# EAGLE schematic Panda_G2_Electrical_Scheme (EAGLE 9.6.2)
AUTHOR: Andrea Maroso; TITLE: Electrical Scheme

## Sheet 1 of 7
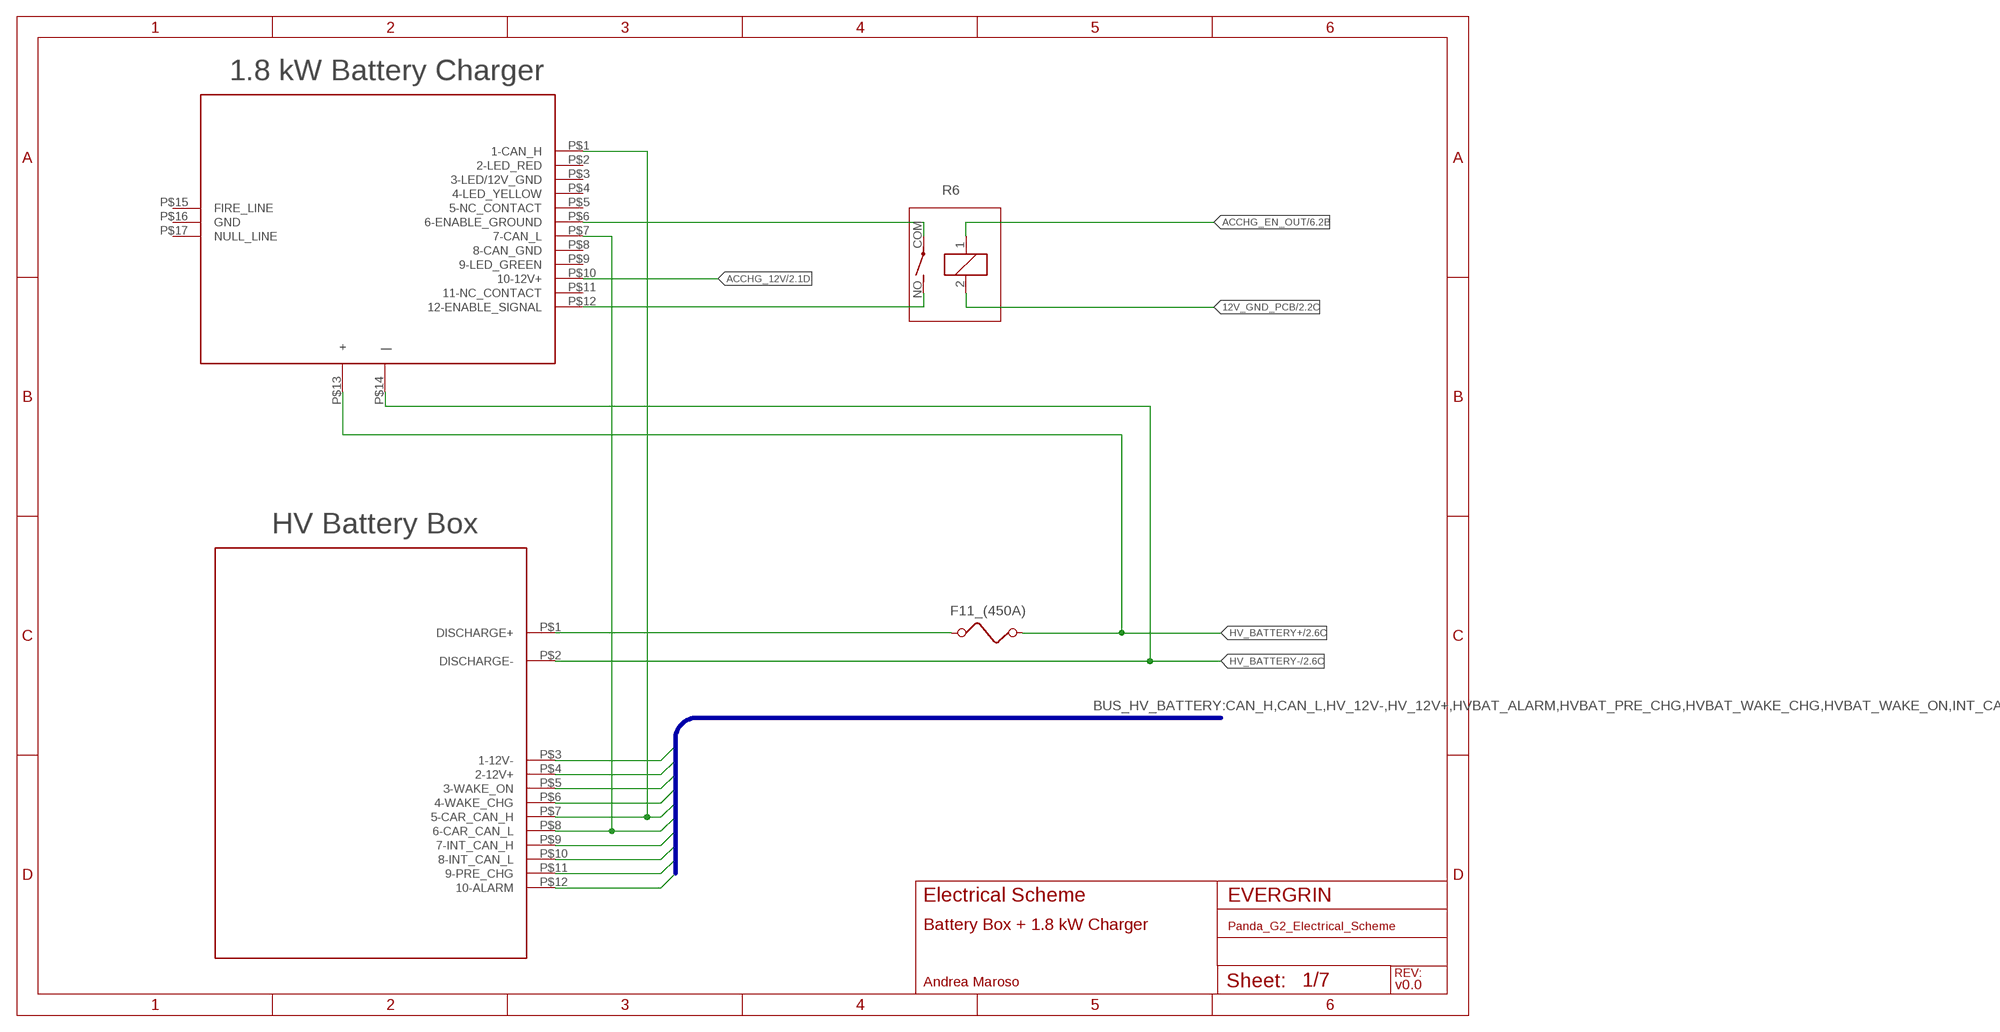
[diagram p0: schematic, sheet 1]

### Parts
F11_(450A)  FUSE  [FUSE]
R6  APF30212A  [APF30212A]
U$1  HV_BATTERY_BOX  [HV_BATTERY_BOX]
U$2  1.8KW_BATTERY_CHARGER  [1.8KW_BATTERY_CHARGER]

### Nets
12V_GND_PCB: R6.2 ; also sheet 2,3,4,5,6,7
ACCHG_12V: U$2.P$10(10-12V+) ; also sheet 2,6
ACCHG_EN_OUT: R6.1 ; also sheet 6
CAN_H: U$1.P$7(5-CAR_CAN_H) U$2.P$1(1-CAN_H) ; also sheet 2,6
CAN_L: U$1.P$8(6-CAR_CAN_L) U$2.P$7(7-CAN_L) ; also sheet 2,6
HV+: F11_(450A).1 U$1.P$1(DISCHARGE+)
HV_12V+: U$1.P$4(2-12V+) ; also sheet 6
HV_12V-: U$1.P$3(1-12V-)
HV_BATTERY+: F11_(450A).2 U$2.P$13(+) ; also sheet 2,4
HV_BATTERY-: U$1.P$2(DISCHARGE-) U$2.P$14(|) ; also sheet 2,4
HVBAT_ALARM: U$1.P$12(10-ALARM) ; also sheet 6
HVBAT_PRE_CHG: U$1.P$11(9-PRE_CHG) ; also sheet 6
HVBAT_WAKE_CHG: U$1.P$6(4-WAKE_CHG) ; also sheet 6
HVBAT_WAKE_ON: U$1.P$5(3-WAKE_ON) ; also sheet 6
INT_CANH: U$1.P$9(7-INT_CAN_H)
INT_CANL: U$1.P$10(8-INT_CAN_L)
N$17: R6.COM(2:P) U$2.P$6(6-ENABLE_GROUND)
N$18: R6.NO(2:S) U$2.P$12(12-ENABLE_SIGNAL)
Unconnected: U$2.P$2(2-LED_RED) U$2.P$3(3-LED/12V_GND) U$2.P$4(4-LED_YELLOW) U$2.P$5(5-NC_CONTACT) U$2.P$8(8-CAN_GND) U$2.P$9(9-LED_GREEN) U$2.P$11(11-NC_CONTACT) U$2.P$15(FIRE_LINE) U$2.P$16(GND) U$2.P$17(NULL_LINE)

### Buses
BUS_HV_BATTERY:CAN_H,CAN_L,HV_12V-,HV_12V+,HVBAT_ALARM,HVBAT_PRE_CHG,HVBAT_WAKE_CHG,HVBAT_WAKE_ON,INT_CANH,INT_CANL

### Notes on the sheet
- Battery Box + 1.8 kW Charger
- v0.0

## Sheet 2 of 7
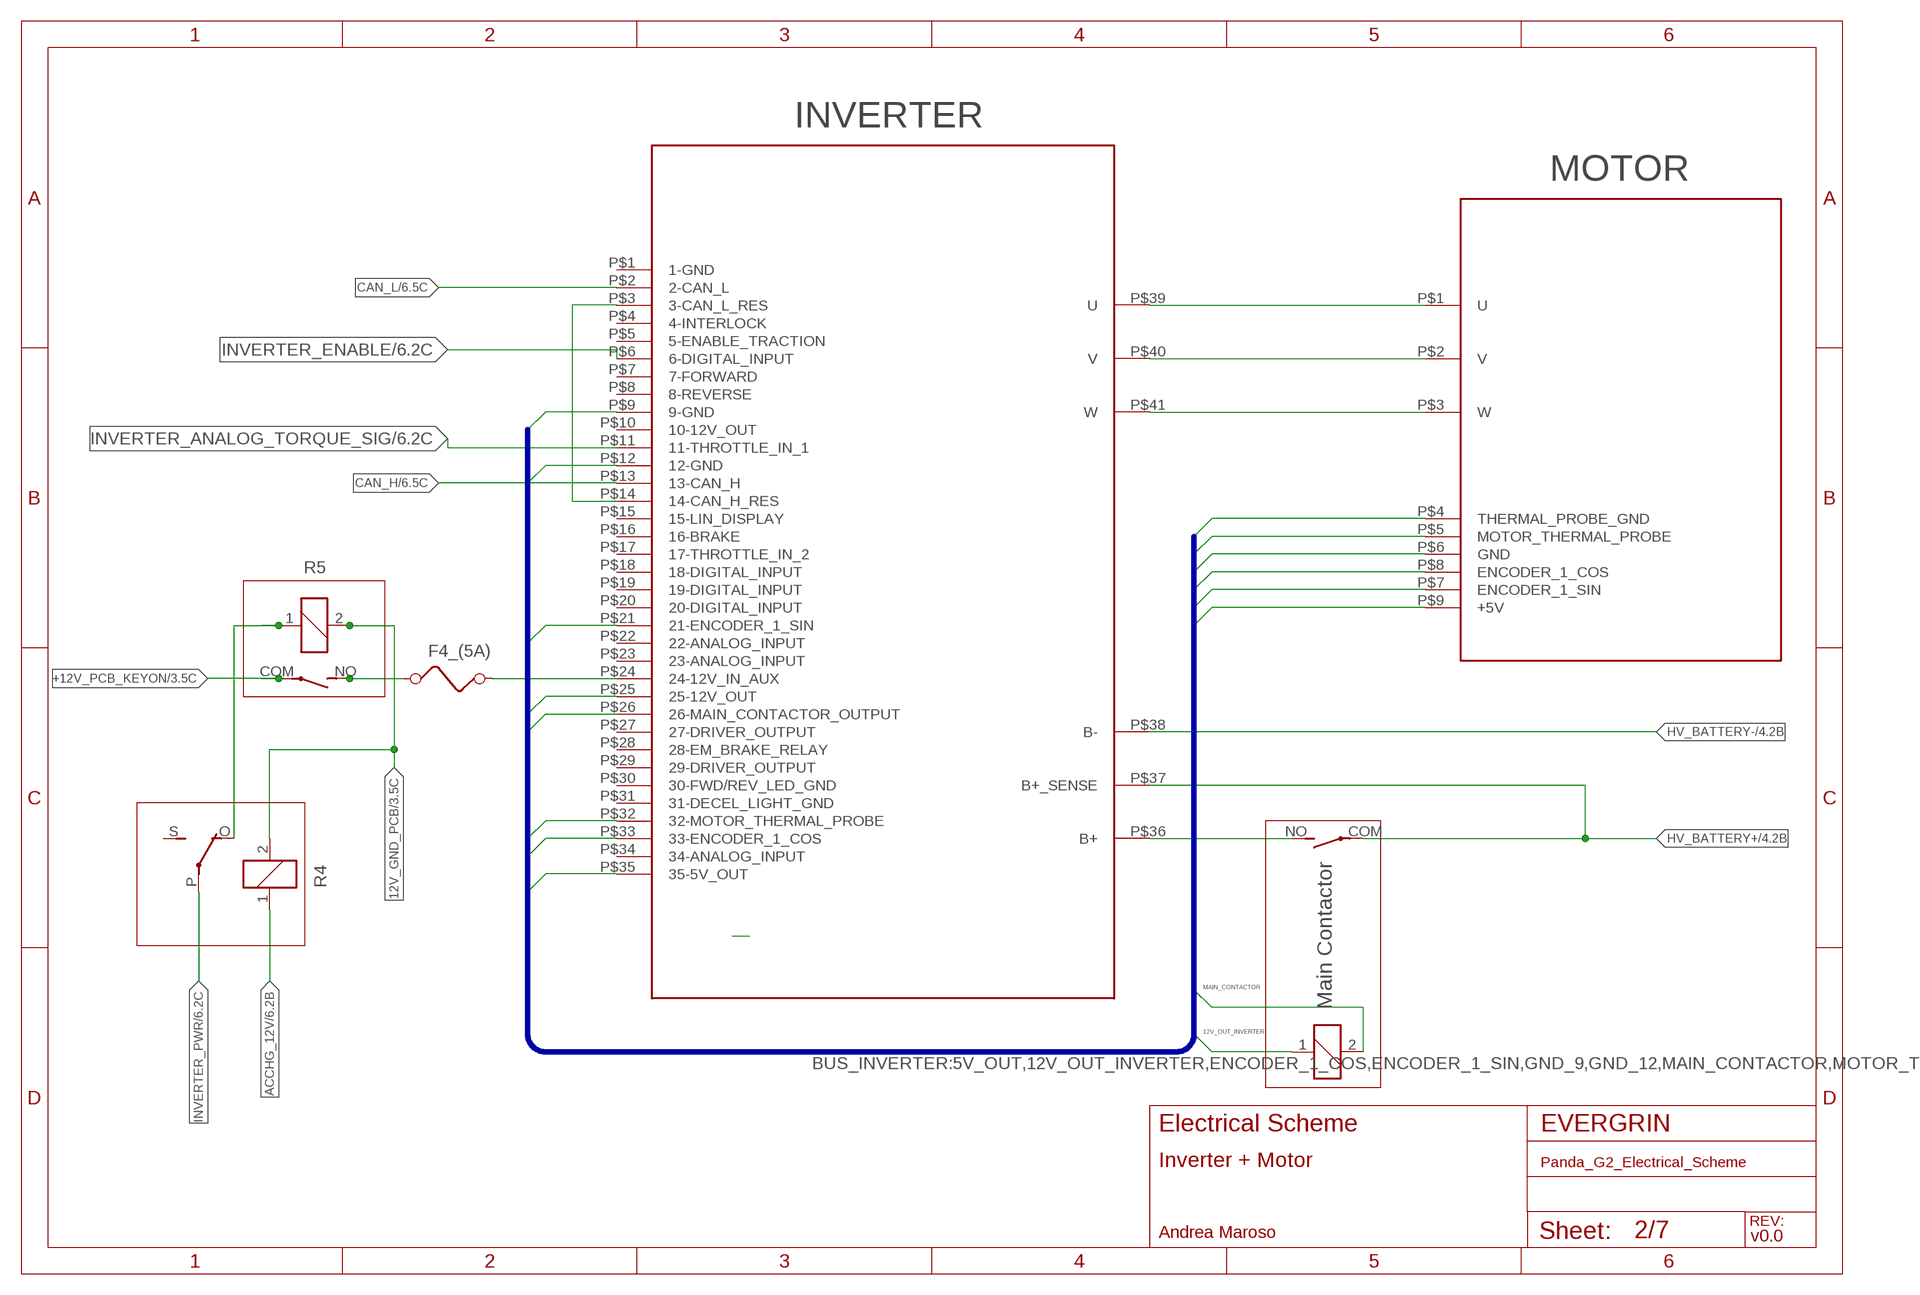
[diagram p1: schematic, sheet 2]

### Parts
F4_(5A)  FUSE  [FUSE]
K1  G5L  [G5LE]
MAIN_CONTACTOR  APF30212A  [APF30212A]
R5  APF30212A  [APF30212A]
U$3  INVERTER  [INVERTER]
U$4  MOTOR  [MOTOR]

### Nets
5V_OUT: U$3.P$35(35-5V_OUT) U$4.P$9(+5V)
12V_GND_PCB: K1.2 R5.2 ; also sheet 1,3,4,5,6,7
12V_OUT_INVERTER: MAIN_CONTACTOR.1 U$3.P$25(25-12V_OUT)
+12V_PCB_KEYON: R5.COM(2:P) ; also sheet 3,5,7
ACCHG_12V: K1.1 ; also sheet 1,6
ACCHG_EN_OUT2: K1.O(2:O) R5.1
CAN_H: U$3.P$13(13-CAN_H) ; also sheet 1,6
CAN_L: U$3.P$2(2-CAN_L) ; also sheet 1,6
ENCODER_1_COS: U$3.P$33(33-ENCODER_1_COS) U$4.P$8(ENCODER_1_COS)
ENCODER_1_SIN: U$3.P$21(21-ENCODER_1_SIN) U$4.P$7(ENCODER_1_SIN)
GND_9: U$3.P$9(9-GND) U$4.P$6(GND)
GND_12: U$3.P$12(12-GND) U$4.P$4(THERMAL_PROBE_GND)
HV_BATTERY+: MAIN_CONTACTOR.COM(2:P) U$3.P$37(B+_SENSE) ; also sheet 1,4
HV_BATTERY-: U$3.P$38(B-) ; also sheet 1,4
INVERTER_ANALOG_TORQUE_SIG: U$3.P$11(11-THROTTLE_IN_1) ; also sheet 6
INVERTER_ENABLE: U$3.P$6(6-DIGITAL_INPUT) ; also sheet 6
INVERTER_PWR: K1.P(2:P) ; also sheet 6
MAIN_CONTACTOR: MAIN_CONTACTOR.2 U$3.P$26(26-MAIN_CONTACTOR_OUTPUT)
MOTOR_THERMAL_PROBE: U$3.P$32(32-MOTOR_THERMAL_PROBE) U$4.P$5(MOTOR_THERMAL_PROBE)
N$1: U$3.P$3(3-CAN_L_RES) U$3.P$14(14-CAN_H_RES)
N$2: U$3.P$39(U) U$4.P$1(U)
N$3: U$3.P$40(V) U$4.P$2(V)
N$4: U$3.P$41(W) U$4.P$3(W)
N$5: MAIN_CONTACTOR.NO(2:S) U$3.P$36(B+)
N$23: F4_(5A).1 R5.NO(2:S)
N$24: F4_(5A).2 U$3.P$24(24-12V_IN_AUX)
Unconnected: K1.S(2:S) U$3.P$1(1-GND) U$3.P$4(4-INTERLOCK) U$3.P$5(5-ENABLE_TRACTION) U$3.P$7(7-FORWARD) U$3.P$8(8-REVERSE) U$3.P$10(10-12V_OUT) U$3.P$15(15-LIN_DISPLAY) U$3.P$16(16-BRAKE) U$3.P$17(17-THROTTLE_IN_2) U$3.P$18(18-DIGITAL_INPUT) U$3.P$19(19-DIGITAL_INPUT) U$3.P$20(20-DIGITAL_INPUT) U$3.P$22(22-ANALOG_INPUT) U$3.P$23(23-ANALOG_INPUT) U$3.P$27(27-DRIVER_OUTPUT) U$3.P$28(28-EM_BRAKE_RELAY) U$3.P$29(29-DRIVER_OUTPUT) U$3.P$30(30-FWD/REV_LED_GND) U$3.P$31(31-DECEL_LIGHT_GND) U$3.P$34(34-ANALOG_INPUT)

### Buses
BUS_INVERTER:5V_OUT,12V_OUT_INVERTER,ENCODER_1_COS,ENCODER_1_SIN,GND_9,GND_12,MAIN_CONTACTOR,MOTOR_THERMAL_PROBE

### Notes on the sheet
- R4 | Main Contactor
- Inverter + Motor
- v0.0

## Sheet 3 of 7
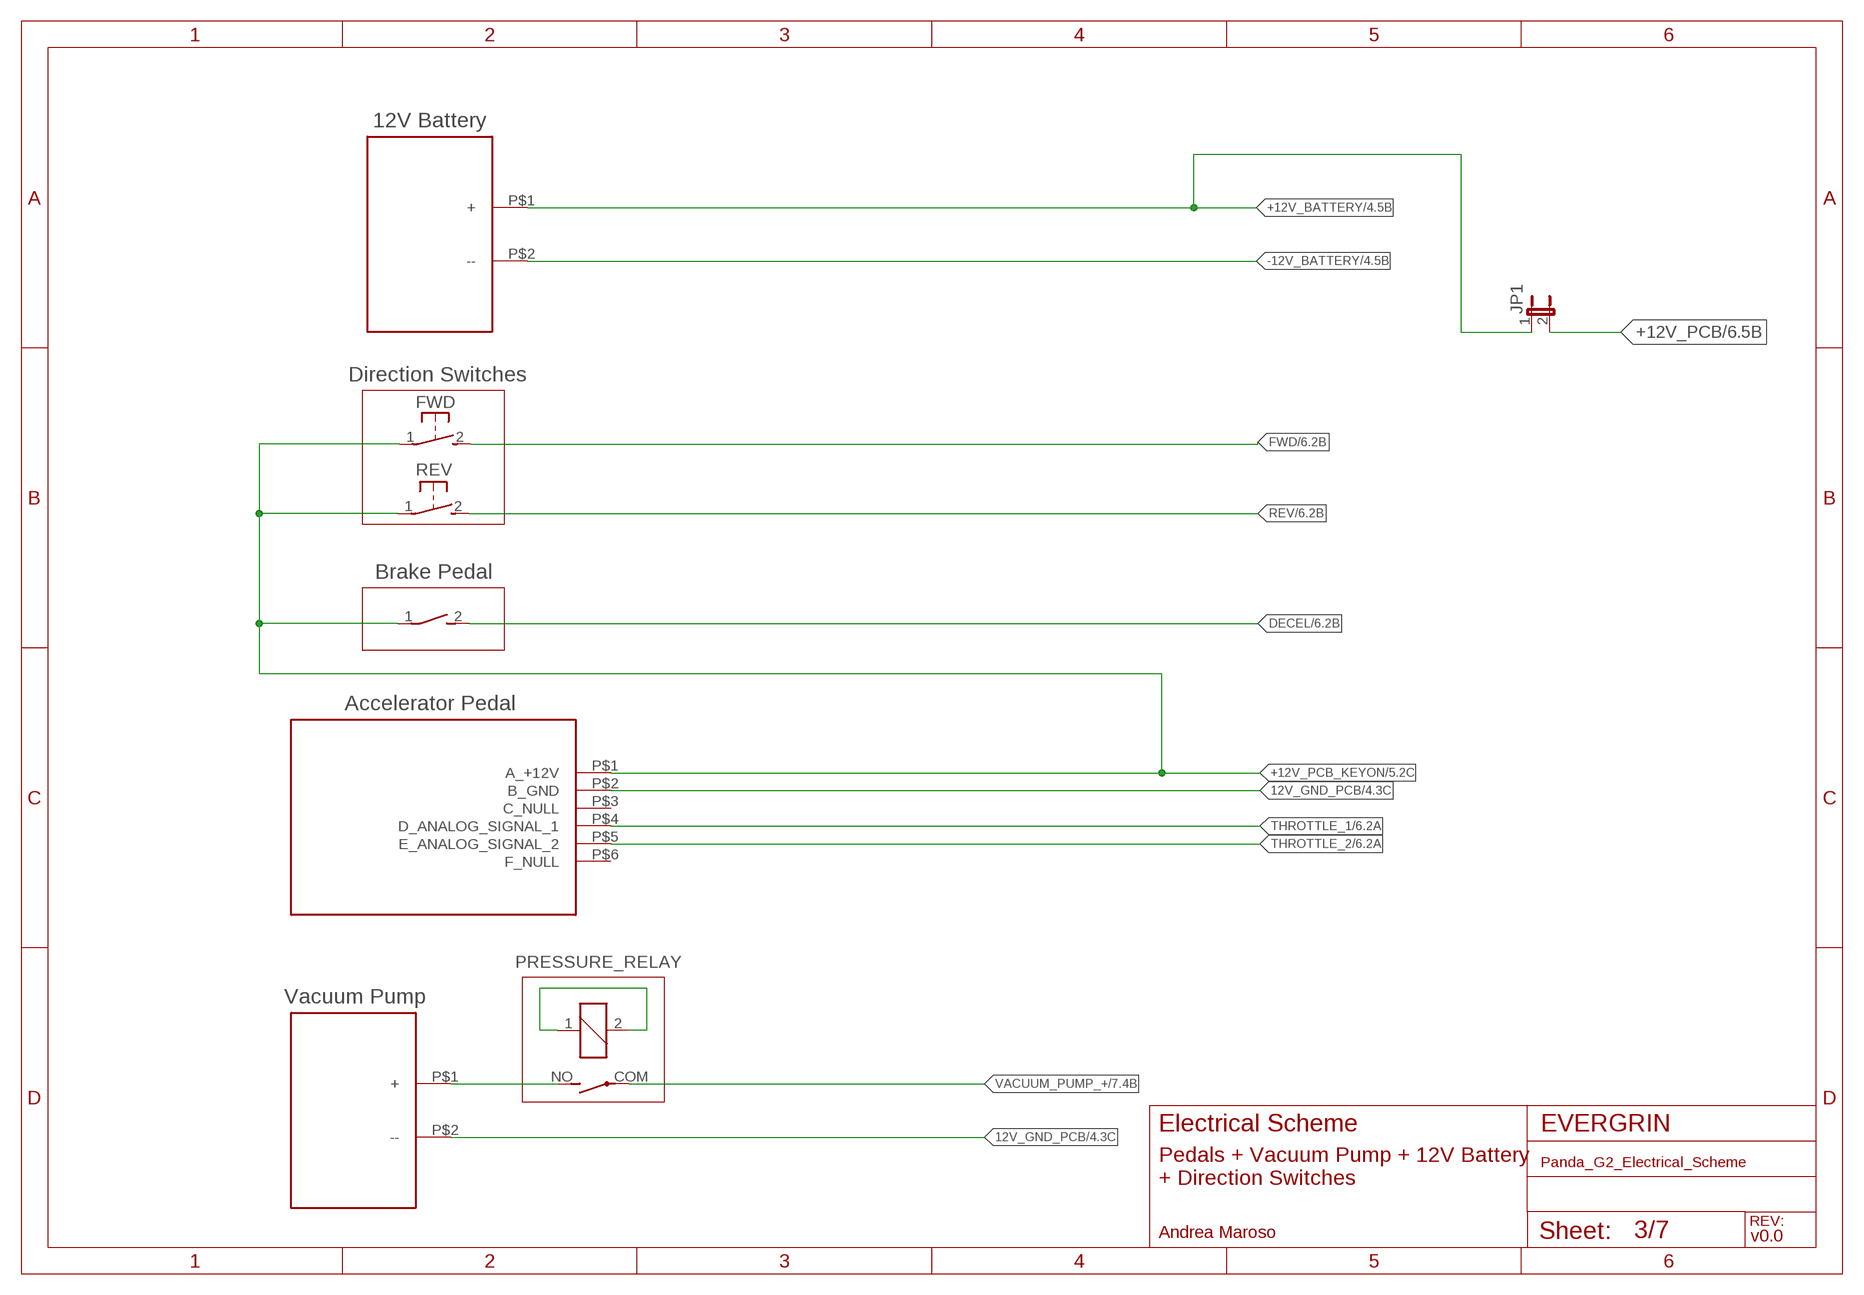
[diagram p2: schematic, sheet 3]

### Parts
JP1  JP1E  [JP1]
PRESSURE_RELAY  APF30212A  [APF30212A]
S1  31-XX  [B3F-31XX]
S2  31-XX  [B3F-31XX]
S4  DS01E  [DS-01]
U$5  12V_BATTERY  [12V_BATTERY]
U$6  ACC_PEDAL  [ACC_PEDAL]
U$7  VACUUM_PUMP  [VACUUM_PUMP]

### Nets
12V_GND_PCB: U$6.P$2(B_GND) U$7.P$2(--) ; also sheet 1,2,4,5,6,7
+12V_BATTERY: JP1.1 U$5.P$1(+) ; also sheet 4,6
+12V_PCB: JP1.2 ; also sheet 6,7
+12V_PCB_KEYON: S1.1(P) S2.1(P) S4.1 U$6.P$1(A_+12V) ; also sheet 2,5,7
-12V_BATTERY: U$5.P$2(--) ; also sheet 4
DECEL: S4.2 ; also sheet 6
FWD: S1.2(S) ; also sheet 6
N$7: PRESSURE_RELAY.1 PRESSURE_RELAY.2
REV: S2.2(S) ; also sheet 6
THROTTLE_1: U$6.P$4(D_ANALOG_SIGNAL_1) ; also sheet 6
THROTTLE_2: U$6.P$5(E_ANALOG_SIGNAL_2) ; also sheet 6
VACUUM_PUMP_+: PRESSURE_RELAY.COM(2:P) PRESSURE_RELAY.NO(2:S) U$7.P$1(+) ; also sheet 7
Unconnected: U$6.P$3(C_NULL) U$6.P$6(F_NULL)

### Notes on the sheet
- Direction Switches
- FWD
- REV
- Brake Pedal
- Pedals + Vacuum Pump + 12V Battery
  + Direction Switches
- v0.0

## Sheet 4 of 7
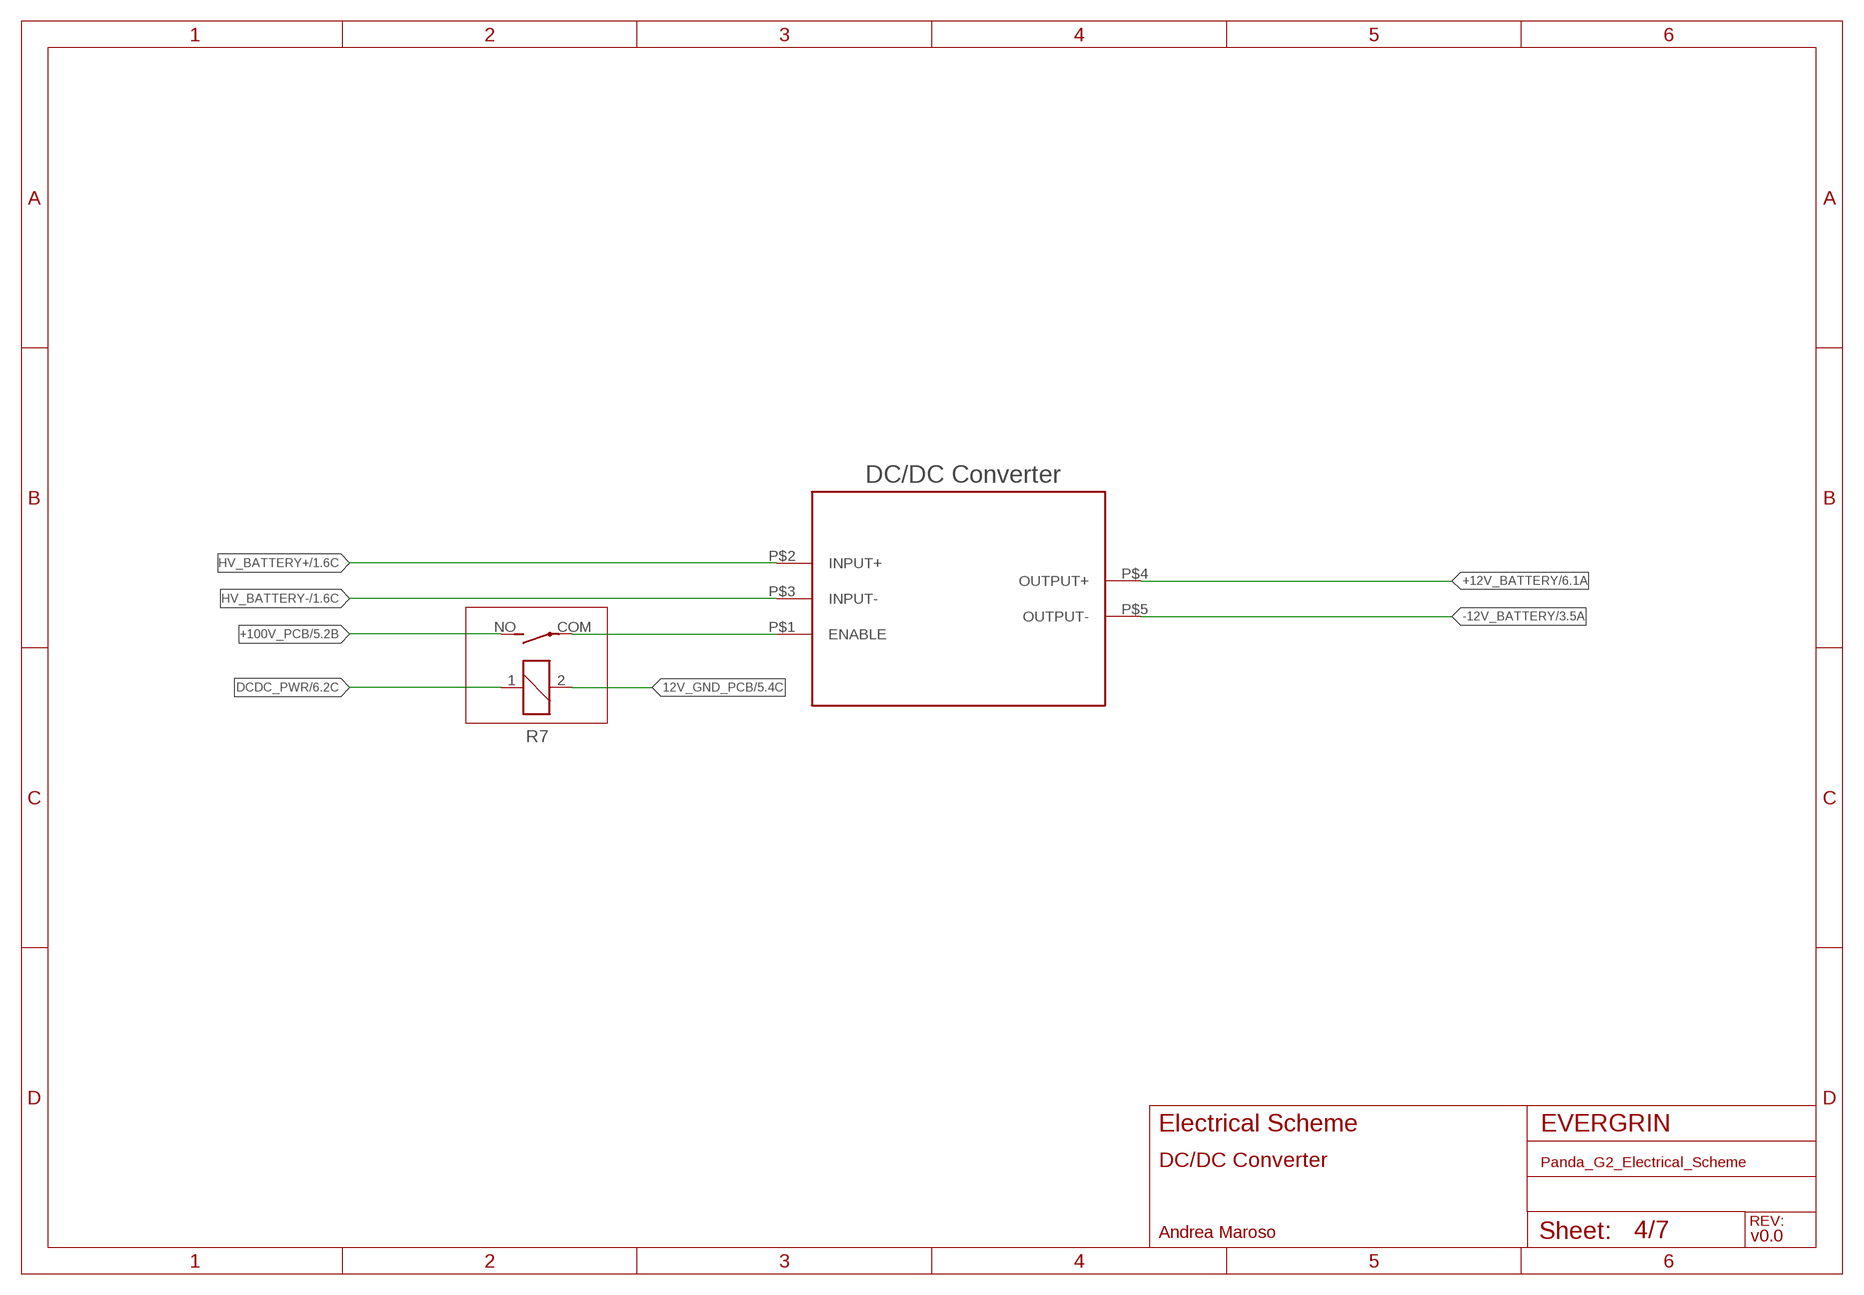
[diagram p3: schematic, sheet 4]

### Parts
R7  APF30212A  [APF30212A]
U$8  DC/DC  [DC/DC]

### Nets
12V_GND_PCB: R7.2 ; also sheet 1,2,3,5,6,7
+12V_BATTERY: U$8.P$4(OUTPUT+) ; also sheet 3,6
+100V_PCB: R7.NO(2:S) ; also sheet 5
-12V_BATTERY: U$8.P$5(OUTPUT-) ; also sheet 3
DCDC_PWR: R7.1 ; also sheet 6
HV_BATTERY+: U$8.P$2(INPUT+) ; also sheet 1,2
HV_BATTERY-: U$8.P$3(INPUT-) ; also sheet 1,2
N$6: R7.COM(2:P) U$8.P$1(ENABLE)

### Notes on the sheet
- DC/DC Converter
- v0.0

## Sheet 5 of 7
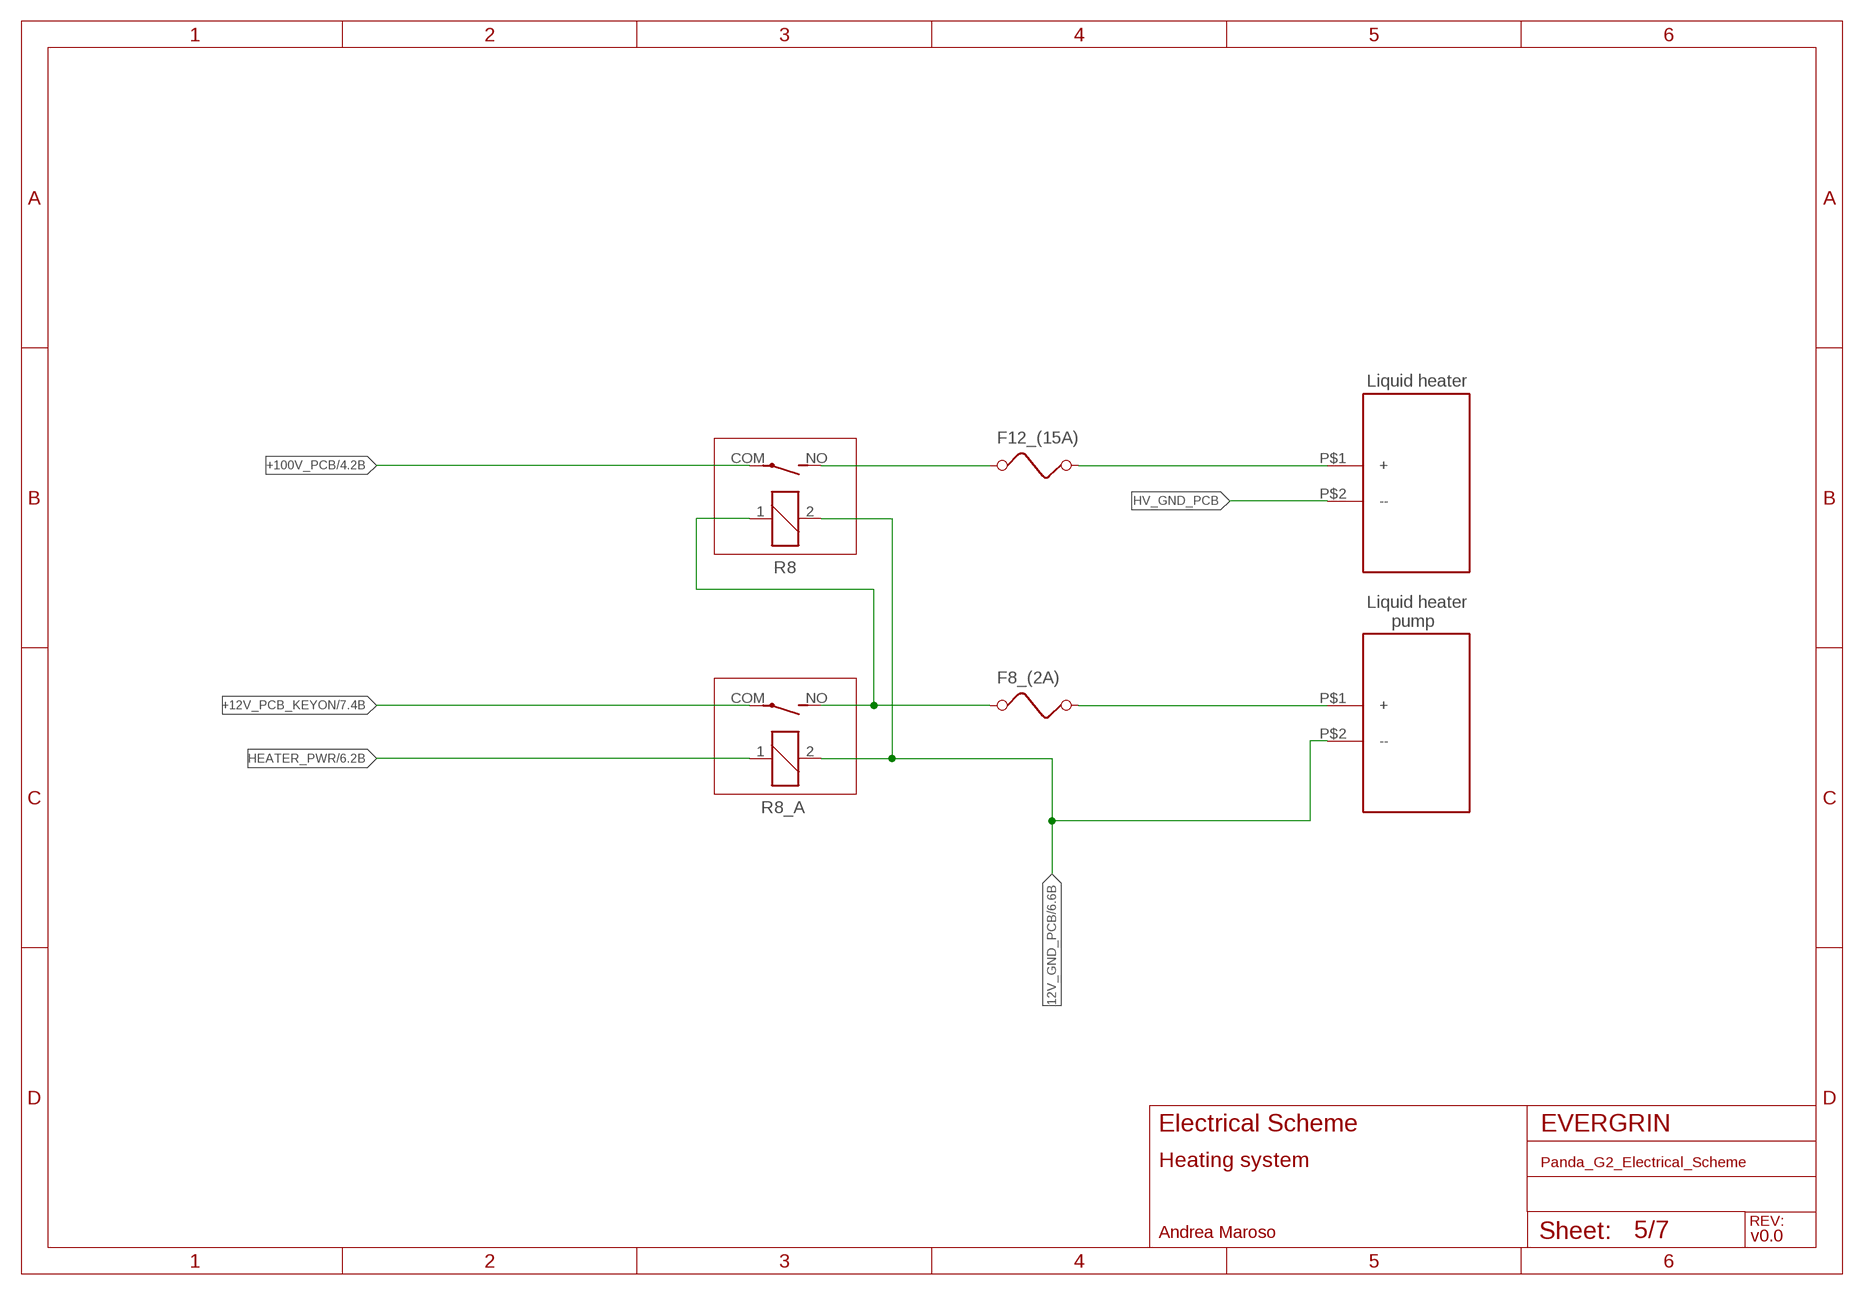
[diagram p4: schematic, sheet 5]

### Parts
F8_(2A)  FUSE  [FUSE]
F12_(15A)  FUSE  [FUSE]
R8  APF30212A  [APF30212A]
R8_A  APF30212A  [APF30212A]
U$9  LIQUID_HEATER  [LIQUID_HEATER]
U$10  LIQUID_HEATER_PUMP  [LIQUID_HEATER_PUMP]

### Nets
12V_GND_PCB: R8.2 R8_A.2 U$10.P$2(--) ; also sheet 1,2,3,4,6,7
+12V_PCB_KEYON: R8_A.COM(2:P) ; also sheet 2,3,7
+100V_PCB: R8.COM(2:P) ; also sheet 4
HEATER_PWR: R8_A.1 ; also sheet 6
HV_GND_PCB: U$9.P$2(--)
N$8: F12_(15A).1 R8.NO(2:S)
N$9: F12_(15A).2 U$9.P$1(+)
N$11: F8_(2A).1 R8.1 R8_A.NO(2:S)
N$12: F8_(2A).2 U$10.P$1(+)

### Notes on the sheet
- Heating system
- v0.0

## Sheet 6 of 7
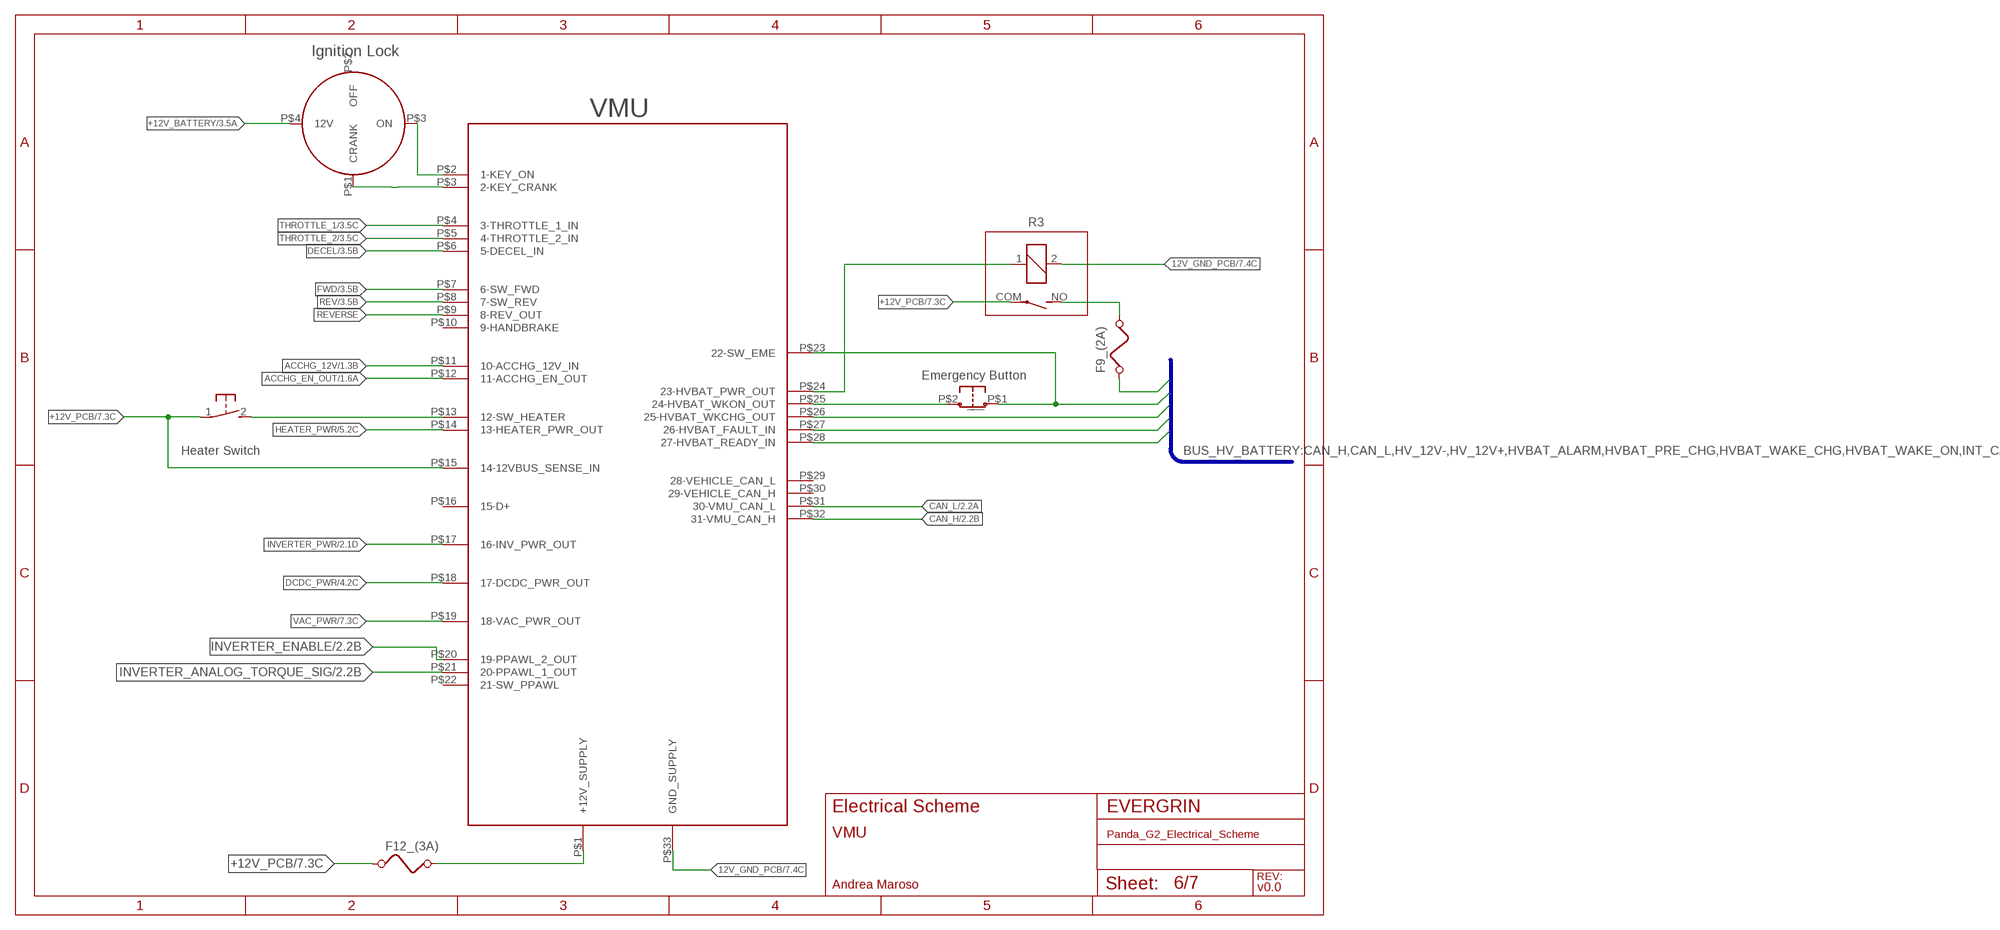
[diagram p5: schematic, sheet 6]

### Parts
F9_(2A)  FUSE  [FUSE]
F12_(3A)  FUSE  [FUSE]
R3  APF30212A  [APF30212A]
S5  31-XX  [B3F-31XX]
U$11  VMU  [VMU]
U$12  IGNITION_LOCK  [IGNITION_LOCK]
U$13  EMERGENCY_BUTTON  [EMERGENCY_BUTTON]

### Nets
12V_GND_PCB: R3.2 U$11.P$33(GND_SUPPLY) ; also sheet 1,2,3,4,5,7
+12V_BATTERY: U$12.P$4(12V) ; also sheet 3,4
+12V_PCB: F12_(3A).1 R3.COM(2:P) S5.1(P) U$11.P$15(14-12VBUS_SENSE_IN) ; also sheet 3,7
ACCHG_12V: U$11.P$11(10-ACCHG_12V_IN) ; also sheet 1,2
ACCHG_EN_OUT: U$11.P$12(11-ACCHG_EN_OUT) ; also sheet 1
CAN_H: U$11.P$32(31-VMU_CAN_H) ; also sheet 1,2
CAN_L: U$11.P$31(30-VMU_CAN_L) ; also sheet 1,2
DCDC_PWR: U$11.P$18(17-DCDC_PWR_OUT) ; also sheet 4
DECEL: U$11.P$6(5-DECEL_IN) ; also sheet 3
FWD: U$11.P$7(6-SW_FWD) ; also sheet 3
HEATER_PWR: U$11.P$14(13-HEATER_PWR_OUT) ; also sheet 5
HV_12V+: F9_(2A).2 ; also sheet 1
HVBAT_ALARM: U$11.P$27(26-HVBAT_FAULT_IN) ; also sheet 1
HVBAT_PRE_CHG: U$11.P$28(27-HVBAT_READY_IN) ; also sheet 1
HVBAT_WAKE_CHG: U$11.P$26(25-HVBAT_WKCHG_OUT) ; also sheet 1
HVBAT_WAKE_ON: U$11.P$23(22-SW_EME) U$13.P$1(_) ; also sheet 1
INVERTER_ANALOG_TORQUE_SIG: U$11.P$21(20-PPAWL_1_OUT) ; also sheet 2
INVERTER_ENABLE: U$11.P$20(19-PPAWL_2_OUT) ; also sheet 2
INVERTER_PWR: U$11.P$17(16-INV_PWR_OUT) ; also sheet 2
KEY_CRANK: U$11.P$3(2-KEY_CRANK) U$12.P$1(CRANK)
KEY_ON: U$11.P$2(1-KEY_ON) U$12.P$3(ON) ; also sheet 7
N$13: U$11.P$25(24-HVBAT_WKON_OUT) U$13.P$2(__)
N$14: F12_(3A).2 U$11.P$1(+12V_SUPPLY)
N$15: R3.1 U$11.P$24(23-HVBAT_PWR_OUT)
N$16: F9_(2A).1 R3.NO(2:S)
N$19: S5.2(S) U$11.P$13(12-SW_HEATER)
REV: U$11.P$8(7-SW_REV) ; also sheet 3
REVERSE: U$11.P$9(8-REV_OUT)
THROTTLE_1: U$11.P$4(3-THROTTLE_1_IN) ; also sheet 3
THROTTLE_2: U$11.P$5(4-THROTTLE_2_IN) ; also sheet 3
VAC_PWR: U$11.P$19(18-VAC_PWR_OUT) ; also sheet 7
Unconnected: U$11.P$10(9-HANDBRAKE) U$11.P$16(15-D+) U$11.P$22(21-SW_PPAWL) U$11.P$29(28-VEHICLE_CAN_L) U$11.P$30(29-VEHICLE_CAN_H) U$12.P$2(OFF)

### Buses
BUS_HV_BATTERY:CAN_H,CAN_L,HV_12V-,HV_12V+,HVBAT_ALARM,HVBAT_PRE_CHG,HVBAT_WAKE_CHG,HVBAT_WAKE_ON,INT_CANH,INT_CANL

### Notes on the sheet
- Heater Switch
- VMU
- v0.0

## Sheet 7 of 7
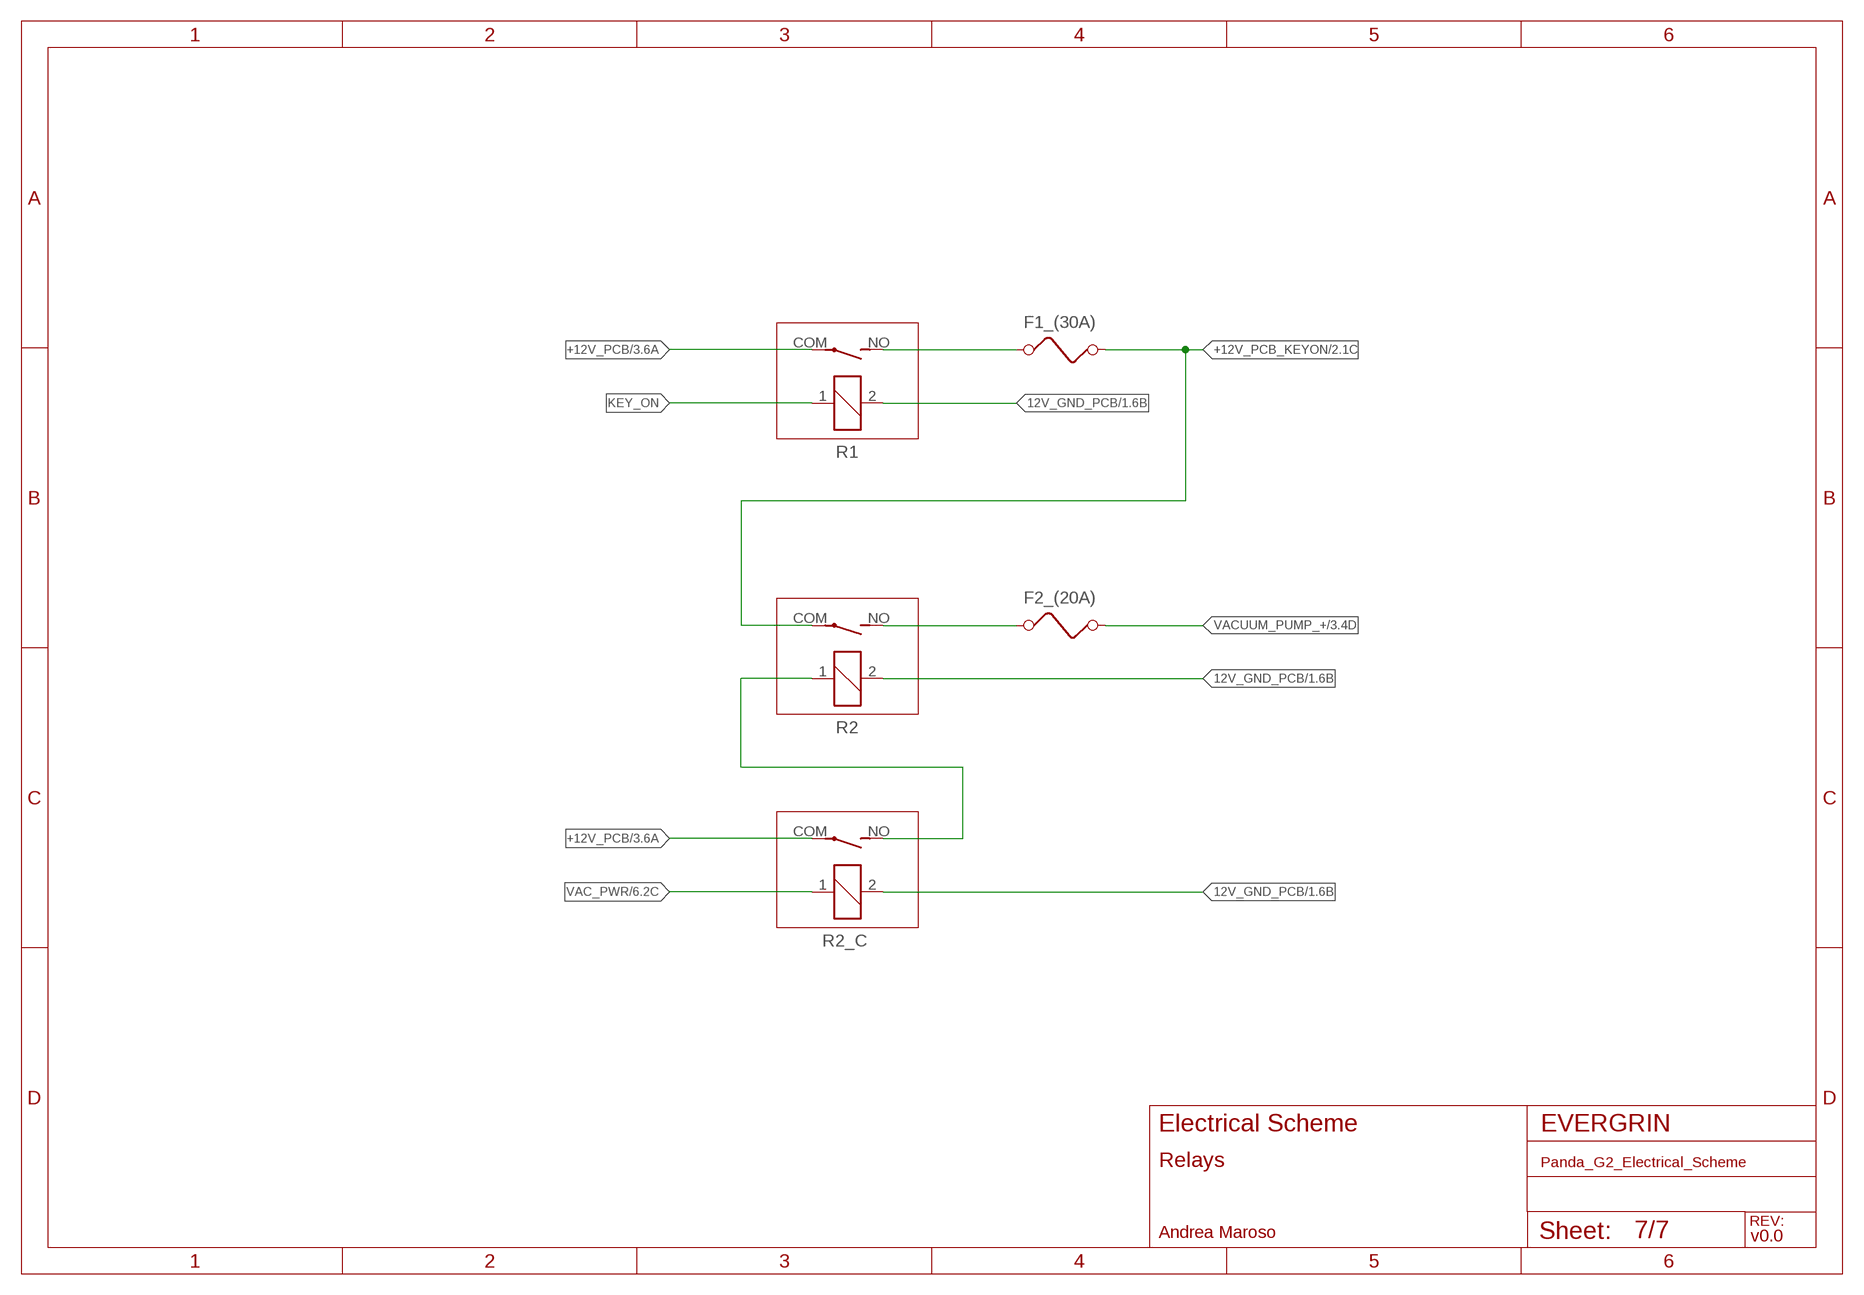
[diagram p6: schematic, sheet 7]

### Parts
F1_(30A)  FUSE  [FUSE]
F2_(20A)  FUSE  [FUSE]
R1  APF30212A  [APF30212A]
R2  APF30212A  [APF30212A]
R2_C  APF30212A  [APF30212A]

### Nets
12V_GND_PCB: R1.2 R2.2 R2_C.2 ; also sheet 1,2,3,4,5,6
+12V_PCB: R1.COM(2:P) R2_C.COM(2:P) ; also sheet 3,6
+12V_PCB_KEYON: F1_(30A).2 R2.COM(2:P) ; also sheet 2,3,5
KEY_ON: R1.1 ; also sheet 6
N$10: F2_(20A).1 R2.NO(2:S)
N$20: F1_(30A).1 R1.NO(2:S)
N$22: R2.1 R2_C.NO(2:S)
VAC_PWR: R2_C.1 ; also sheet 6
VACUUM_PUMP_+: F2_(20A).2 ; also sheet 3

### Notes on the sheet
- Relays
- v0.0

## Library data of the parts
F1_(30A) F2_(20A) F4_(5A) F8_(2A) F9_(2A) F11_(450A) F12_(3A) F12_(15A) = special:FUSE: FUSE
JP1 = jumper:JP1E: JUMPER
K1 = relay:G5L: RELAY 1 x switch, 10 A/120 V AC, 8 A/30 V ADC, Omron; OC_FARNELL: unknown; OC_NEWARK: unknown
MAIN_CONTACTOR PRESSURE_RELAY R1 R2 R2_C R3 R5-R8 R8_A = relay:APF30212A: Compliant with European standards 1a/1c 6A Slim power relays Source: Data sheet; OC_FARNELL: unknown
S1 S2 S5 = switch-omron:31-XX: OMRON SWITCH; MPN: B3F-3100; OC_FARNELL: 959704; OC_NEWARK: 36M3582
S4 = switch-dil:DS01E: DIL/CODE SWITCH; OC_FARNELL: unknown; OC_NEWARK: unknown
U$1 = EVERGRIN_Panda_G2:HV_BATTERY_BOX: HV battery box
U$2 = EVERGRIN_Panda_G2:1.8KW_BATTERY_CHARGER: 1.8 kW battery charger
U$3 = EVERGRIN_Panda_G2:INVERTER: Inverter
U$4 = EVERGRIN_Panda_G2:MOTOR: Motor
U$5 = EVERGRIN_Panda_G2:12V_BATTERY: 12 V battery
U$6 = EVERGRIN_Panda_G2:ACC_PEDAL: Accelerator pedal
U$7 = EVERGRIN_Panda_G2:VACUUM_PUMP
U$8 = EVERGRIN_Panda_G2:DC/DC
U$9 = EVERGRIN_Panda_G2:LIQUID_HEATER: Liquid Heater
U$10 = EVERGRIN_Panda_G2:LIQUID_HEATER_PUMP: Liquid Heater Pump
U$11 = EVERGRIN_Panda_G2:VMU
U$12 = EVERGRIN_Panda_G2:IGNITION_LOCK
U$13 = EVERGRIN_Panda_G2:EMERGENCY_BUTTON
